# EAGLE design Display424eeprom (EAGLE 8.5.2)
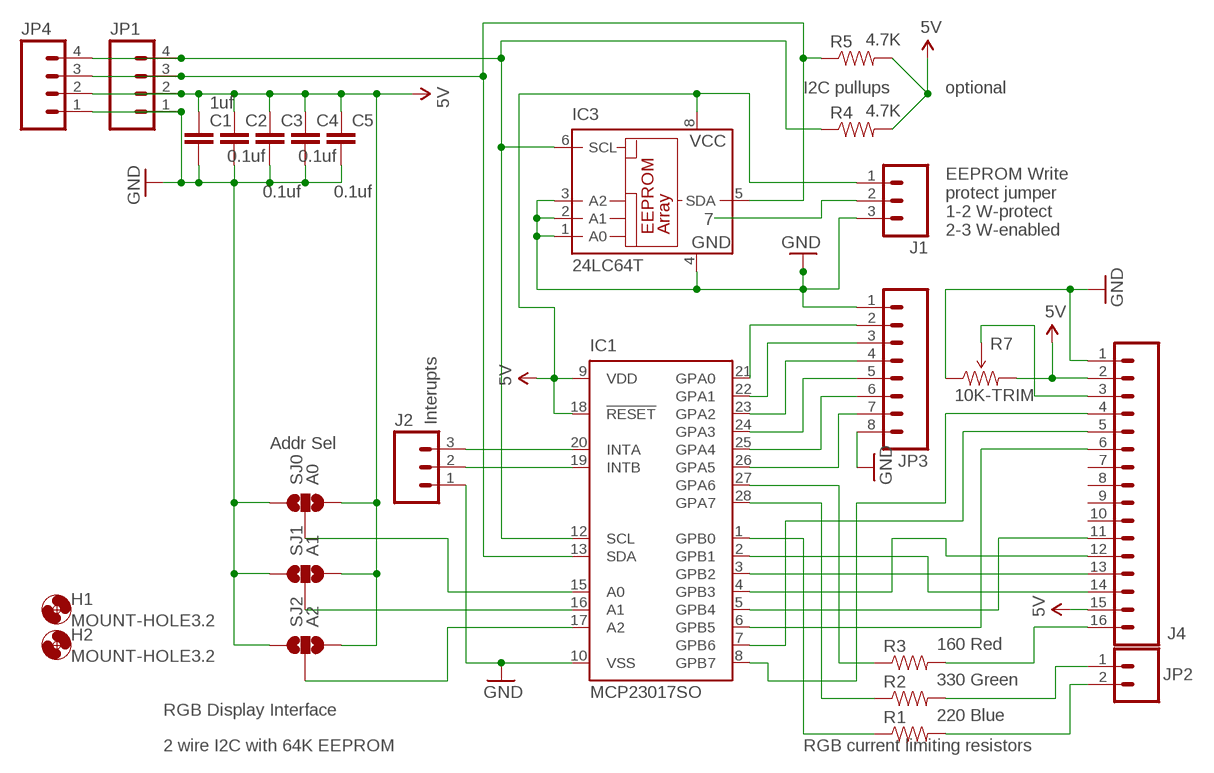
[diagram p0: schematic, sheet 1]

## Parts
C1  1uf  CAPEZ  [CAP-PTH-SMALLEZ]
C2  0.1uf  CAPEZ  [CAP-PTH-SMALLEZ]
C3  0.1uf  CAPEZ  [CAP-PTH-SMALLEZ]
C4  0.1uf  CAPEZ  [CAP-PTH-SMALLEZ]
C5  0.1uf  CAPEZ  [CAP-PTH-SMALLEZ]
H1  MOUNT-HOLE3.2  [3,2]
H2  MOUNT-HOLE3.2  [3,2]
IC1  MCP23017SO  [SO28W]
IC3  24LC64T  24-LC65SM  [SO-08M]
J1  M03LOCK  [1X03_LOCK]
J2  M03LOCK  [1X03_LOCK]
J4  M16LOCK  [1X16_LOCK]
JP1  M04LOCK_LONGPADS  [1X04_LOCK_LONGPADS]
JP2  M02PTH  [1X02]
JP3  M08LOCK  [1X08_LOCK]
JP4  M04LOCK_LONGPADS  [1X04_LOCK_LONGPADS]
R1  220 Blue  RESISTORPTH-1/4W  [AXIAL-0.4]
R2  330 Green  RESISTORPTH-1/4W  [AXIAL-0.4]
R3  160 Red  RESISTORPTH-1/4W  [AXIAL-0.4]
R4  4.7K  RESISTORKIT  [AXIAL-0.3-KIT]
R5  4.7K  RESISTORKIT  [AXIAL-0.3-KIT]
R7  10K-TRIM  TRIMPOT-2  [TRIMPOT_TC33]
SJ0  A0  SOLDERJUMPER_2WAYPASTE2&3  [SJ_3_PASTE2&3]
SJ1  A1  SOLDERJUMPER_2WAYPASTE2&3  [SJ_3_PASTE2&3]
SJ2  A2  SOLDERJUMPER_2WAYPASTE2&3  [SJ_3_PASTE2&3]

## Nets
5V: C1.1 C2.1 C3.1 C4.1 C5.1 IC1.9(VDD) IC1.18(!RESET) IC3.8(VCC) J1.1 J4.2 J4.15 JP1.2 JP4.2 R4.P$2 R5.P$2 R7.3(CW) SJ0.3 SJ1.3 SJ2.3
GND: C1.2 C2.2 C3.2 C4.2 C5.2 IC1.10(VSS) IC3.1(A0) IC3.2(A1) IC3.3(A2) IC3.4(GND) J1.3 J2.1 J4.1 JP1.1 JP3.1 JP3.8 JP4.1 R7.1(CCW) SJ0.1 SJ1.1 SJ2.1
N$1: IC1.1(GPB0) R1.P$1
N$2: JP2.2 R1.P$2
N$3: IC1.28(GPA7) R2.P$1
N$4: JP2.1 R2.P$2
N$5: IC1.27(GPA6) R3.P$1
N$6: J4.16 R3.P$2
N$7: IC1.2(GPB1) J4.14
N$8: IC1.3(GPB2) J4.13
N$9: IC1.4(GPB3) J4.12
N$10: IC1.5(GPB4) J4.11
N$11: IC1.6(GPB5) J4.6
N$12: IC1.7(GPB6) J4.5
N$13: IC1.8(GPB7) J4.4
N$14: J4.3 R7.2(WIPER)
N$17: J1.2
N$18: IC1.21(GPA0) JP3.2
N$19: IC1.23(GPA2) JP3.4
N$20: IC1.24(GPA3) JP3.5
N$21: IC1.22(GPA1) JP3.3
N$22: IC1.16(A1) SJ1.2
N$24: IC1.15(A0) SJ0.2
N$25: IC1.25(GPA4) JP3.6
N$26: IC1.26(GPA5) JP3.7
N$27: IC1.17(A2) SJ2.2
N$28: IC1.20(INTA) J2.3
N$29: IC1.19(INTB) J2.2
SCL: IC1.12(SCL) IC3.6(SCL) JP1.4 JP4.4 R4.P$1
SDA: IC1.13(SDA) IC3.5(SDA) JP1.3 JP4.3 R5.P$1
Unconnected: J4.7 J4.8 J4.9 J4.10

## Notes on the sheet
- I2C pullups | optional
- 7
- EEPROM Write
  protect jumper
  1-2 W-protect
  2-3 W-enabled
- Interupts
- Addr Sel
- RGB Display Interface
- 2 wire I2C with 64K EEPROM | RGB current limiting resistors

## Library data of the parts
C1-C5 = SparkFun-Capacitors:CAP: Capacitor
H1 H2 = holes:MOUNT-HOLE: MOUNTING HOLE with drill center marker
IC1 = adafruit:MCP23017: http://ww1.microchip.com/downloads/en/DeviceDoc/21952a.pdf Source: http://ww1.microchip.com/downloads/en/DeviceDoc/21952a.pdf
IC3 = microchip:24-*: Serial EEPROM 32 K/64 K, 1.8 V, I2C; MF: MICROCHIP; MPN: 24LC65/SM; OC_FARNELL: 9758097; OC_NEWARK: 96K4082
J1 J2 = SparkFun-Connectors:M03: Header 3 Standard 3-pin 0.1" header. Use with straight break away headers (SKU : PRT-00116), right angle break away headers (PRT-00553), swiss pins (PRT-00743), machine pins (PRT-00117), and female headers (PRT-00115). Molex polarized connector foot print use with SKU : PRT-08232 with associated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
J4 = SparkFun-Connectors:M16: 1x16 .1" header
JP1 JP4 = SparkFun-Connectors:M04: Header 4 Standard 4-pin 0.1" header. Use with straight break away headers (SKU : PRT-00116), right angle break away headers (PRT-00553), swiss pins (PRT-00743), machine pins (PRT-00117), and female headers (PRT-00115). Molex polarized connector foot print use with SKU : PRT-08231 with associated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
JP2 = SparkFun-Connectors:M02: Standard 2-pin 0.1" header. Use with
JP3 = SparkFun-Connectors:M08: Header 8 Standard 8-pin 0.1" header. Use with straight break away headers (SKU : PRT-00116), right angle break away headers (PRT-00553), swiss pins (PRT-00743), machine pins (PRT-00117), and female headers (PRT-00115).
R1-R5 = SparkFun-Resistors:RESISTOR: Resistor
R7 = SparkFun-Electromechanical:TRIMPOT: Various small potentiometers for "set-and-forget" applications
SJ0 SJ1 SJ2 = SparkFun-Passives:SOLDERJUMPER_2WAY: Solder Jumper 2 way solder jumper

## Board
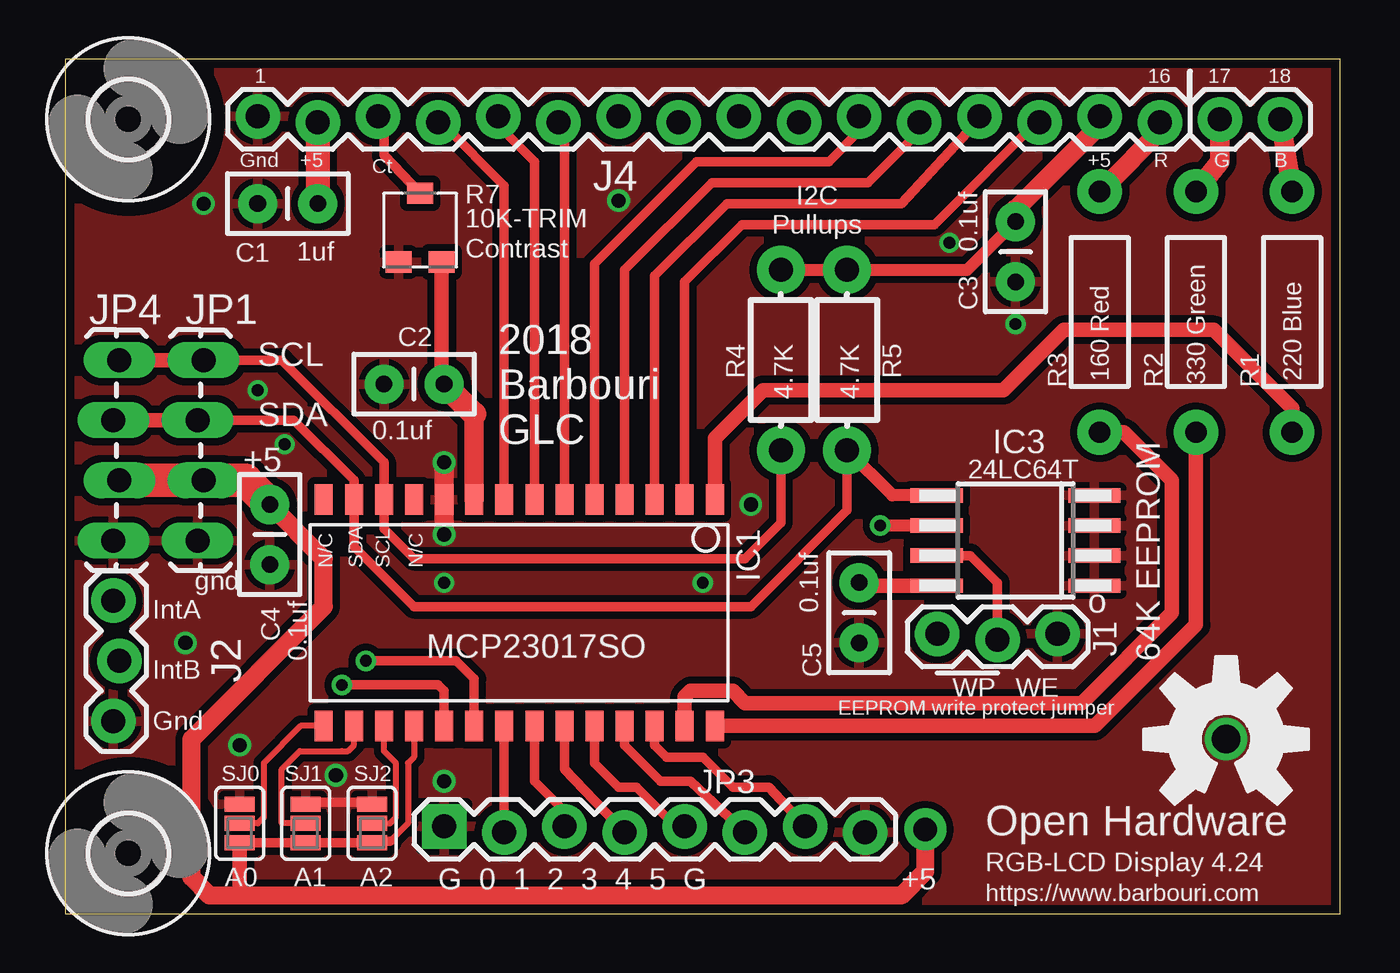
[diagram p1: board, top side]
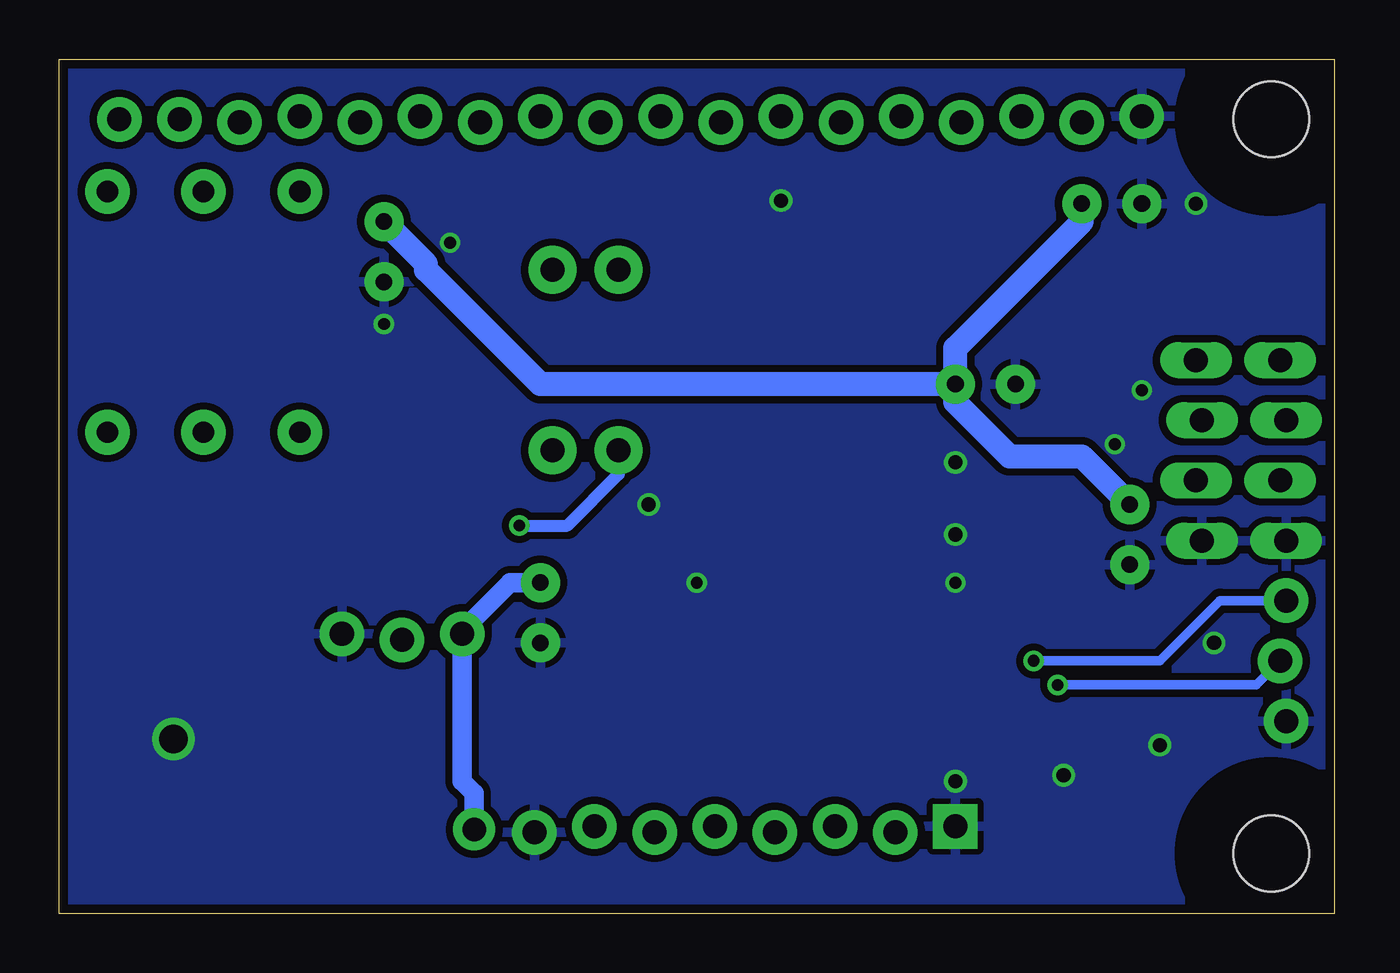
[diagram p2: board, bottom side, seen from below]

Size 53.85 x 36.07 mm. Coordinates in mm from the lower left corner, seen from the top.
Outline: 0,0 53.85,0 53.85,36.07 0,36.07 0,0
Copper layers (1*16): Top 0.0356mm / dielectric 1.5011mm / Bottom 0.0356mm
Design rules "default *": minimum track width 10mil, minimum drill 13mil, track to track 12mil, track to pad 12mil, pad to pad 12mil, via to via 10mil, smd to smd 6mil, copper to edge 15mil, drill to drill 8mil, minimum pad ring 7mil, minimum via ring 7mil, stop-mask expansion 4mil, vias tented up to drill 24mil, thermal gap 10mil

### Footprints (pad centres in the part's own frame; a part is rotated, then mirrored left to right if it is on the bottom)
CAP-PTH-SMALLEZ = drill 0.7 pad 1.651: 1 0,0; 2 2.54,0
3,2 = hole 3.2: 0,0
SO28W = smd 0.762 x 1.27: 1 -7.62,-4.78; 2 -6.35,-4.78; 3 -5.08,-4.78; 4 -3.81,-4.78; 5 -2.54,-4.78; 6 -1.27,-4.78; 7 0,-4.78; 8 1.27,-4.78; 9 2.54,-4.78; 10 3.81,-4.78; 11 5.08,-4.78; 12 6.35,-4.78; 13 7.62,-4.78; 14 8.89,-4.78; 15 8.89,4.78; 16 7.62,4.78; 17 6.35,4.78; 18 5.08,4.78; 19 3.81,4.78; 20 2.54,4.78; 21 1.27,4.78; 22 0,4.78; 23 -1.27,4.78; 24 -2.54,4.78; 25 -3.81,4.78; 26 -5.08,4.78; 27 -6.35,4.78; 28 -7.62,4.78
SO-08M = smd 0.6 x 2.2: 1 -1.905,-3.33; 2 -0.635,-3.33; 3 0.635,-3.33; 4 1.905,-3.33; 5 1.905,3.33; 6 0.635,3.33; 7 -0.635,3.33; 8 -1.905,3.33
1X03_LOCK = drill 1.016 pad 1.88: 1 0,0.127; 2 2.54,-0.127; 3 5.08,0.127
1X16_LOCK = drill 1.016 pad 1.88: 1 0,0.127; 2 2.54,-0.127; 3 5.08,0.127; 4 7.62,-0.127; 5 10.16,0.127; 6 12.7,-0.127; 7 15.24,0.127; 8 17.78,-0.127; 9 20.32,0.127; 10 22.86,-0.127; 11 25.4,0.127; 12 27.94,-0.127; 13 30.48,0.127; 14 33.02,-0.127; 15 35.56,0.127; 16 38.1,-0.127
1X04_LOCK_LONGPADS = drill 1.016 long: 1 0,0; 2 2.54,-0.254; 3 5.08,0; 4 7.62,-0.254
1X02 = drill 1.016 pad 1.88: 1 0,0; 2 2.54,0
1X08_LOCK = drill 1.016 pad 1.88 square: 1 0,0.127 | drill 1.016 pad 1.88: 2 2.54,-0.127; 3 5.08,0.127; 4 7.62,-0.127; 5 10.16,0.127; 6 12.7,-0.127; 7 15.24,0.127; 8 17.78,-0.127
AXIAL-0.4 = drill 0.9 pad 1.88: P$1 -5.08,0; P$2 5.08,0
AXIAL-0.3-KIT = drill 1.016 pad 2.032: P$1 -3.81,0; P$2 3.81,0
TRIMPOT_TC33 = smd 1.1 x 0.9: 1 -0.91,-1.45; 2 0,1.45; 3 0.91,-1.45
SJ_3_PASTE2&3 = smd 0.635 x 1.27: 1 -0.813,0; 2 0,0; 3 0.813,0

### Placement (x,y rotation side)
C1  10.67,29.97 180 top
C2  16,22.35 180 top
C3  40.13,29.21 270 top
C4  8.64,17.27 270 top
C5  33.53,13.97 270 top
H1  2.67,33.53 0 top
H2  2.67,2.54 0 top
IC1  19.81,12.7 180 top
IC3  40.13,15.75 90 top
J1  36.83,11.68 0 top
J2  2.16,8.13 90 top
J4  8.13,33.53 0 top
JP1  5.59,15.75 90 top
JP2  48.77,33.53 0 top
JP3  16,3.56 0 top
JP4  2.03,15.75 90 top
R1  51.82,25.4 90 top
R2  47.75,25.4 90 top
R3  43.69,25.4 90 top
R4  30.23,23.37 90 top
R5  33.02,23.37 90 top
R7  14.99,28.96 0 top
SJ0  7.37,3.81 270 top
SJ1  10.16,3.81 270 top
SJ2  12.95,3.81 270 top
U$1  [OSHW-LOGO-L]  49.02,7.37 0 top

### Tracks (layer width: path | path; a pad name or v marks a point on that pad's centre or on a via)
5V  (via drill 1 pad 1.78)
  Top 0.254: IC1.18 14.73,6.6 14.48,6.35 14.48,3.81 13.72,3.05 | 13.01,3.05 SJ2.3
  Top 0.305: J4.15 43.69,33.27
  Top 0.406: SJ0.3 SJ1.3 SJ2.3 | 13.72,3.05 13.01,3.05 | 15.9,22.46 C2.1 | J4.2 10.67,33.53 | J4.15
  Top 0.508: C3.1 38.1,27.18 R5.P$2 R4.P$2
  Top 0.61: C3.1 40.13,28.96 | SJ0.3 7.37,0.76 | R7.3 15.9,22.46 | IC3.8 33.91,13.84 C5.1
  Top 0.762: C4.1 10.92,14.99 10.92,12.95 5.33,7.37 5.33,1.52 6.1,0.76 7.37,0.76 35.31,0.76 36.32,1.78 v36.32,3.56
  Top 0.813: 40.13,29.72 43.69,33.27 | 17.27,21.08 IC1.9
  Top 0.864: C3.1 40.13,29.72
  Top 0.914: 10.67,33.53 J4.2
  Top 1.016: J4.2 C1.1 | C2.1 17.27,21.08
  Top 1.422: C4.1 7.62,18.29 JP1.2 JP4.2
  Bottom 0.61: J1.1 36.83,11.94
  Bottom 0.813: v36.32,3.56 36.32,5.08 36.83,5.59 J1.1 | 36.83,11.94 34.8,13.97 C5.1
  Bottom 1.016: C4.1 10.67,19.3 13.72,19.3 16,21.59 C2.1 | C2.1 33.53,22.35 38.35,27.18 38.35,27.43 C3.1 | C2.1 16,23.88 10.67,29.21 C1.1
GND  (via drill 0.5, 0.6, 1.2)
  Top 0.406: 10.16,4.7 12.95,4.7 13.08,4.57
  Top 0.813: v16,19.05 v16,16
  other vias: 37.34,28.32 28.96,17.27 11.43,5.84 23.37,30.1 5.84,29.97 49.02,7.37 16,5.59 7.37,7.11 8.13,22.1 9.27,19.81 40.13,24.89 5.08,11.43 16,13.97 26.92,13.97
  pour Top: 0,0 53.85,0 53.85,36.07 0,36.07
  pour Bottom: 0,0 53.85,0 53.85,36.07 0,36.07
N$1
  Top 0.61: R1.P$1 51.82,21.34 48.51,24.64 42.16,24.64 39.62,22.1 29.46,22.1 27.43,20.07 IC1.1
N$2
  Top 0.813: JP2.2 R1.P$2
N$3
  Top 0.61: IC1.28 43.48,7.92 47.75,12.19 R2.P$1
N$4
  Top 0.813: R2.P$2 48.77,31.75 JP2.1
N$5
  Top 0.61: IC1.27 26.16,9.14 26.42,9.4 28.19,9.4 28.7,8.89 42.93,8.89 46.74,12.7 46.74,18.29 44.7,20.32 R3.P$1
N$6
  Top 0.406: 46.48,33.27 J4.16
  Top 0.813: 46.48,33.27 R3.P$2
N$7
  Top 0.406: IC1.2 26.16,26.67 28.57,29.08 36.7,29.08 41.15,33.53 J4.14
N$8
  Top 0.305: J4.13 38.61,33.53
  Top 0.406: IC1.3 24.89,26.92 27.94,29.97 35.31,29.97 38.61,33.53 | J4.13
N$9
  Top 0.406: IC1.4 23.62,27.18 27.3,30.86 33.91,30.86 35.81,32.77 35.81,33.15 J4.12
N$10
  Top 0.406: IC1.5 22.35,27.43 26.67,31.75 32.26,31.75 33.53,33.02 J4.11 33.53,33.54
N$11
  Top 0.305: J4.6 20.95,33.41 21.08,33.27
  Top 0.406: 21.08,33.53 21.08,33.27 IC1.6 | J4.6
N$12
  Top 0.305: J4.5 18.42,33.65 18.54,33.02
  Top 0.406: IC1.7 19.81,31.75 18.54,33.02 | J4.5
N$13
  Top 0.305: J4.4 15.88,33.41 16,33.27
  Top 0.406: IC1.8 18.54,30.73 16,33.27 | J4.4
N$14
  Top 0.305: 13.21,33.54 13.45,33.54 13.46,33.53
  Top 0.406: R7.2 13.46,32 13.46,33.53 | J4.3 13.21,33.54
N$18
  Top 0.406: JP3.2 IC1.21
N$19
  Top 0.406: JP3.4 21.08,6.1 IC1.23
N$20
  Top 0.406: JP3.5 25.91,3.56 24.13,5.33 23.37,5.33 22.35,6.35 IC1.24
N$21
  Top 0.406: JP3.3 21.08,4.32 19.81,5.59 IC1.22
N$22
  Top 0.254: 9.91,3.81 SJ1.2 9.91,3.81 | 9.91,3.81 9.14,3.81 9.14,6.1 9.91,6.86 11.68,6.86 11.94,6.86 12.19,7.11 IC1.16
N$24
  Top 0.254: IC1.15 9.95,7.92 8.38,6.35 8.38,4.06 8.13,3.81 SJ0.2 7.11,3.81
N$25
  Top 0.406: IC1.25 23.62,7.11 25.15,5.59 26.42,5.59 JP3.6
N$26
  Top 0.406: IC1.26 24.89,7.11 25.4,6.6 26.92,6.6 28.19,5.33 29.72,5.33 JP3.7
N$27
  Top 0.254: IC1.17 13.46,6.86 13.97,6.35 13.97,4.06 13.72,3.81 SJ2.2 12.7,3.81
N$28  (via drill 0.5)
  Top 0.406: IC1.20 17.27,9.91 16.51,10.67 v12.7,10.67
  Bottom 0.406: v12.7,10.67 7.37,10.67 4.83,13.21 J2.3
N$29  (via drill 0.5)
  Top 0.406: IC1.19 16,9.4 15.75,9.65 v11.68,9.65
  Bottom 0.406: v11.68,9.65 3.3,9.65 J2.2
N$30
  Top 0.406: 36.7,15.11 38.23,15.11 39.37,13.97 39.37,11.68
SCL  (via drill 0.5)
  Top 0.406: JP1.4 9.14,23.37 13.46,19.05 IC1.12 13.46,16.26 14.73,14.99 28.7,14.99 30.23,16.51 R4.P$1
  Top 0.508: IC3.6 v34.42,16.38
  Top 0.61: JP4.4 JP1.4
  Bottom 0.508: v34.42,16.38 32.38,16.38 30.23,18.54 R4.P$1
SDA
  Top 0.406: JP1.3 9.65,20.83 12.19,18.29 IC1.13 12.19,15.49 14.73,12.95 28.96,12.95 33.02,17.02 R5.P$1
  Top 0.508: IC3.5 34.92,17.65 R5.P$1
  Top 0.61: JP4.3 JP1.3

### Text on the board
tNames: 1 | 16 | 17 | 18 | Gnd | +5 | Ct | +5 | R | G | B | I2C / Pullups | Contrast | SCL | SDA | +5 | 2018 / Barbouri / GLC | N/C | SDA | SCL | N/C | gnd | o | IntA | 64K EEPROM | IntB | WP | WE | Gnd | EEPROM write protect jumper | Open Hardware | RGB-LCD Display 4.24 | G 0 1 2 3 4 5 G | +5 | https://www.barbouri.com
